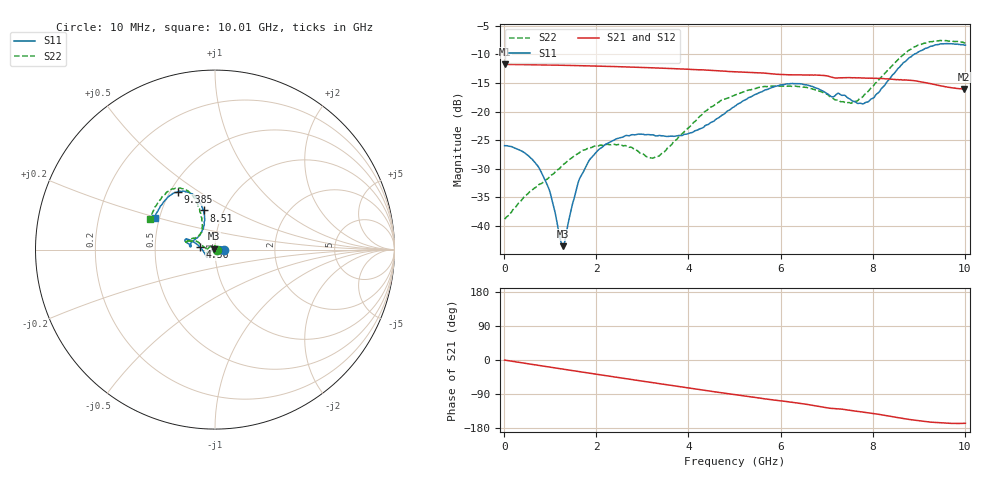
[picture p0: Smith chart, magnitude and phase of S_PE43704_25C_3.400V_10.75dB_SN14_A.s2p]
! Device ID: PE43704
! Dir: z:\PE43704\PE43704_Char_1_20130516\PE43704\AMB\3p400V\10p75dB
! Serial: 14
! Insertion: A
! Impedance: 50 ohm
! Temp: Amb
! VDD: 3.400V
! Attenuation Step: 10.75dB
! IDD: 1.140268e-01mA
#  Hz  S  RI  R  50
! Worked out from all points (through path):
!   401 points, 10 MHz to 10.01 GHz, reference 50 ohm
!   highest |S21| = -11.75 dB at 10 MHz (marker M1); lowest = -16.1 dB at 9.985 GHz (marker M2)
!   group delay of S21, straight-line fit = 48.2 ps
!   lowest |S11| = -43.5 dB at 1.285 GHz (marker M3), VSWR 1.01, Z = 49.6 + j0.53 ohm
!   |S11| at or under -10 dB: start of sweep to 8.898 GHz
!   |S22| runs from -38.8 to -7.6 dB; largest |S21 - S12| = 0.0019
!   S11 on the Smith chart (normalised r, x): 10 MHz: 1.11, +0.00; 4.56 GHz: 0.85, +0.02; 8.51 GHz: 0.81, +0.37; 9.385 GHz: 0.55, +0.41; 10.01 GHz: 0.47, +0.20
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1e7  0.0502 0.000126  0.2584 -0.000963  0.2585 -0.000893  0.0114 0.000357
4.35e8  0.042 0.0125  0.2536 -0.0372  0.254 -0.0374  0.00597 0.0169
7.6e8  0.0274 0.0166  0.2476 -0.0638  0.2475 -0.0637  -0.0061 0.0222
9.85e8  0.0144 0.0143  0.2415 -0.0814  0.2415 -0.0813  -0.0165 0.0212
1.21e9  0.000576 0.00793  0.234 -0.0986  0.234 -0.0986  -0.0279 0.0156
1.285e9  -0.00395 0.00534  0.2311 -0.1041  0.2312 -0.104  -0.0318 0.0132
1.685e9  -0.0254 -0.012  0.2141 -0.1322  0.2142 -0.132  -0.0452 -0.00272
2.01e9  -0.0367 -0.0254  0.1977 -0.1526  0.1977 -0.1523  -0.0476 -0.0143
2.385e9  -0.0425 -0.0368  0.1762 -0.1735  0.1764 -0.1734  -0.0472 -0.0209
3.36e9  -0.0493 -0.0371  0.1116 -0.2122  0.112 -0.212  -0.0406 -0.00333
4.01e9  -0.0633 -0.0123  0.0647 -0.2246  0.065 -0.2246  -0.0695 0.0209
4.56e9  -0.0817 0.0125  0.0246 -0.2267  0.0251 -0.2267  -0.1034 0.0468
5.01e9  -0.1061 0.0336  -0.00519 -0.2226  -0.00487 -0.2226  -0.1311 0.0473
5.96e9  -0.1582 0.0588  -0.0622 -0.202  -0.0617 -0.2022  -0.1593 0.0474
6.685e9  -0.1609 0.0407  -0.1017 -0.1816  -0.102 -0.1815  -0.1495 0.0503
7.56e9  -0.1091 0.0577  -0.1363 -0.1426  -0.1364 -0.1429  -0.0801 0.0892
7.885e9  -0.0773 0.0931  -0.1483 -0.1281  -0.1478 -0.1288  -0.0705 0.1297
8.36e9  -0.0584 0.1826  -0.1631 -0.1015  -0.1627 -0.1023  -0.0853 0.2207
8.51e9  -0.0628 0.2179  -0.1664 -0.091  -0.1661 -0.0922  -0.0975 0.2562
9.385e9  -0.2087 0.3217  -0.1649 -0.0436  -0.1653 -0.0427  -0.2505 0.3294
9.985e9  -0.3308 0.1875  -0.1532 -0.0346  -0.1532 -0.0345  -0.3561 0.1784
1.001e10  -0.3365 0.1775  -0.1538 -0.0353  -0.1544 -0.0354  -0.3602 0.1703
